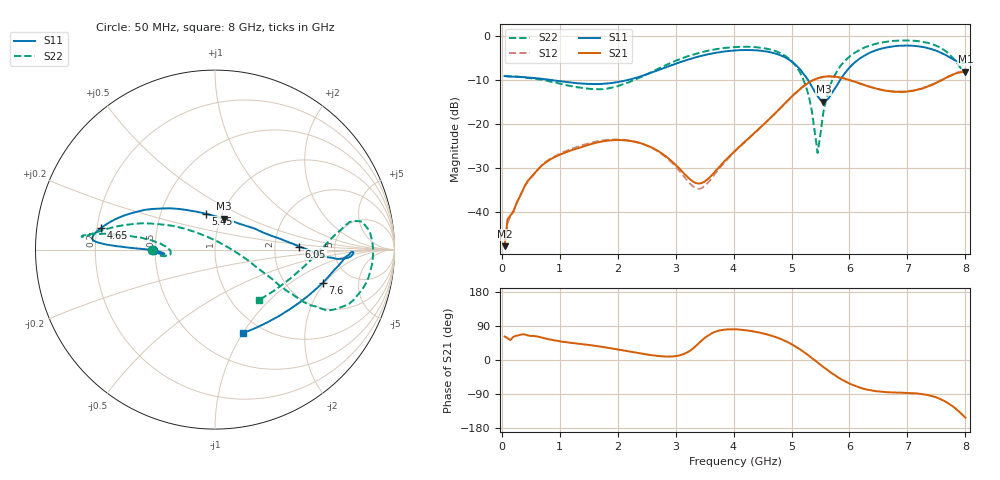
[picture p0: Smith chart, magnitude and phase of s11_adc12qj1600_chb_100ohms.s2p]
#  HZ  S  DB  R  100.00
! Rohde & Schwarz ZVA24 4Ports - Version 4.10 - 1145.1110k26 SN: 100644
! Date: 2020-07-21 15:20:36
! Measurements: S11 S31 S13 S33
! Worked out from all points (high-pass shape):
!   160 points, 50 MHz to 8 GHz, reference 100 ohm
!   highest |S21| = -8.17 dB at 8 GHz (marker M1); lowest = -47.7 dB at 50 MHz (marker M2)
!   |S21| within 3 dB of the highest: 5.239 GHz to 6.255 GHz (1.015 GHz wide, 17.7 % of centre); 7.422 GHz to end of sweep
!   lowest |S11| = -14.9 dB at 5.55 GHz (marker M3), VSWR 1.44, Z = 103 + j36.9 ohm
!   |S11| at or under -10 dB: 822.1 MHz to 2.192 GHz (1.37 GHz wide, 90.9 % of centre); 5.281 GHz to 5.841 GHz (559.8 MHz wide, 10.1 % of centre)
!   |S22| runs from -26.6 to -1.1 dB; largest |S21 - S12| = 0.015
!   S11 on the Smith chart (normalised r, x): 50 MHz: 0.48, -0.00; 4.65 GHz: 0.22, +0.09; 5.45 GHz: 0.84, +0.35; 6.05 GHz: 2.77, +0.12; 7.6 GHz: 3.14, -1.91; 8 GHz: 0.82, -1.00
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5e7  -9.17 -179.5  -47.66 62.1  -47.11 61.3  -9.11 -179.7
1e8  -9.24 -180.0  -41.60 57.8  -42.52 58.0  -9.19 -179.4
4.5e8  -9.49 -177.9  -32.89 64.9  -33.01 65.4  -9.60 -176.5
8e8  -9.96 -176.2  -28.35 55.1  -28.20 56.6  -10.29 -173.6
1.4e9  -10.87 -174.7  -25.11 41.6  -24.76 41.1  -11.86 -173.5
2.1e9  -10.28 -177.7  -23.68 25.0  -23.58 22.7  -10.97 175.8
2.7e9  -7.82 179.5  -26.13 10.6  -26.25 7.3  -7.48 170.8
3.4e9  -4.73 177.7  -33.49 44.1  -34.71 44.7  -3.92 172.1
4.05e9  -3.34 175.6  -25.75 80.9  -25.88 83.7  -2.58 174.0
4.65e9  -3.81 169.1  -18.47 64.3  -18.51 66.4  -3.21 172.7
5.1e9  -6.97 150.4  -12.67 32.9  -12.71 34.8  -7.32 160.1
5.25e9  -9.37 137.4  -11.08 17.1  -11.13 19.1  -11.48 150.4
5.35e9  -11.51 124.3  -10.22 5.3  -10.27 7.3  -16.98 137.4
5.45e9  -13.72 104.1  -9.67 -6.4  -9.71 -4.5  -26.57 66.4
5.55e9  -14.93 74.6  -9.33 -18.6  -9.38 -16.6  -17.31 -10.9
5.7e9  -12.93 34.7  -9.27 -35.4  -9.31 -33.3  -10.17 -25.7
6.05e9  -6.56 2.0  -10.29 -65.5  -10.30 -63.5  -4.24 -30.3
6.7e9  -2.55 -3.4  -12.60 -85.5  -12.54 -83.1  -1.28 -12.3
7.3e9  -2.66 -2.7  -11.77 -90.9  -11.68 -88.5  -1.51 10.1
7.6e9  -4.02 -17.0  -10.08 -105.6  -9.97 -103.3  -3.01 8.8
7.8e9  -5.45 -38.2  -8.75 -124.3  -8.65 -122.1  -5.26 -5.2
8e9  -6.18 -71.5  -8.17 -152.3  -8.05 -150.3  -8.57 -49.3
